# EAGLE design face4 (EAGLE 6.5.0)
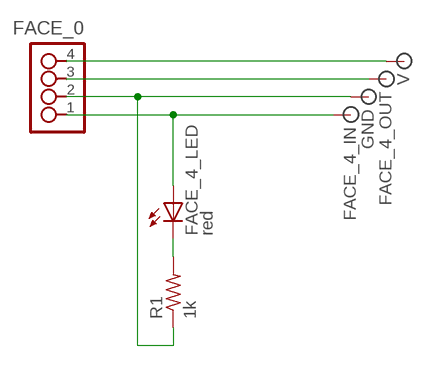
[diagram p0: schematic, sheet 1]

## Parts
FACE_0  4_PIN_HEADER  [SMT_PINS_4]
FACE_4_IN  SIGNAL  [PAD.2]
FACE_4_LED  red  LED1206  [1206]
FACE_4_OUT  SIGNAL  [PAD.2]
GND  SIGNAL  [PAD.2]
R1  1k  RESISTOR1206  [1206]
V  SIGNAL  [PAD.2]

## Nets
N$1: FACE_0.2 GND.P$1 R1.1
N$2: FACE_0.1 FACE_4_IN.P$1 FACE_4_LED.1(A)
N$4: FACE_0.3 FACE_4_OUT.P$1
N$5: FACE_4_LED.2(C) R1.2
N$6: FACE_0.4 V.P$1

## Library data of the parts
FACE_0 = ot:4_PIN_HEADER
FACE_4_IN FACE_4_OUT GND V = ot:SIGNAL: Signal
FACE_4_LED = 01_FAB_Hello:LED
R1 = 01_FAB_Hello:RESISTOR

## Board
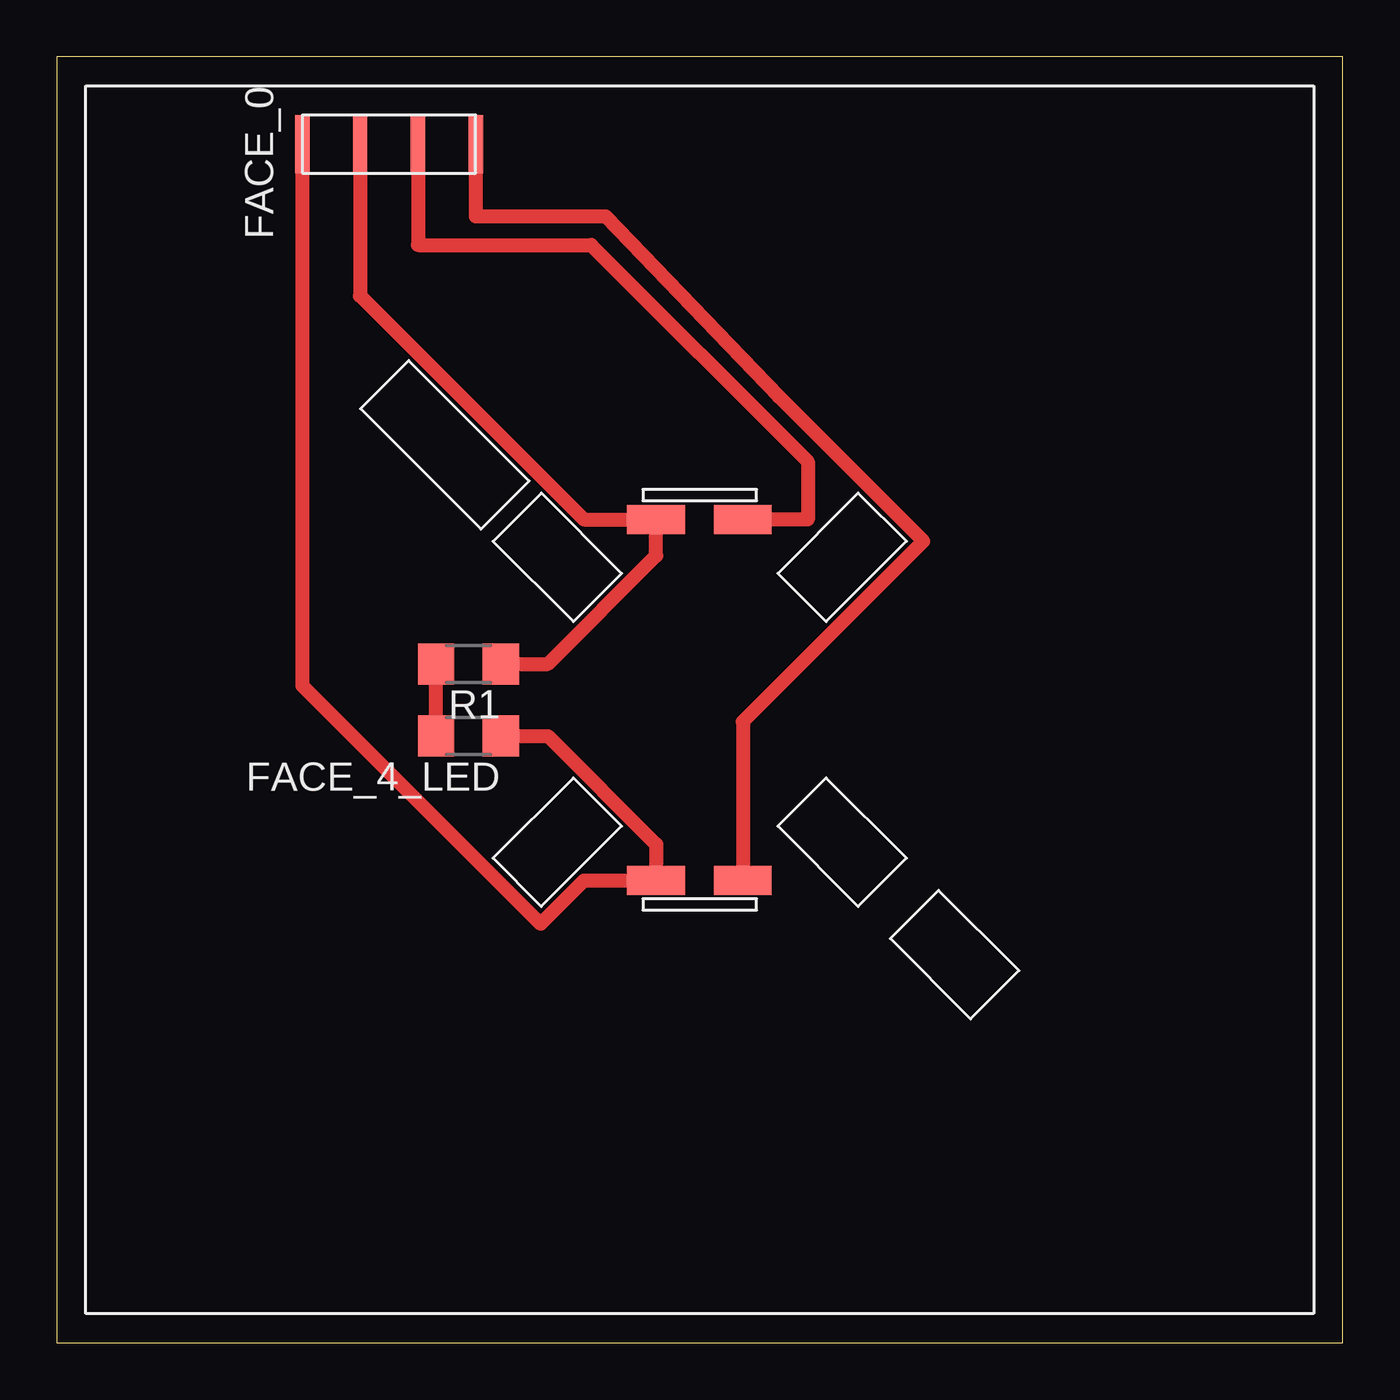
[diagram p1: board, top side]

Size 56.54 x 56.54 mm. Coordinates in mm from the lower left corner, seen from the top.
Outline: 0,0 56.54,0 56.54,56.54 0,56.54 0,0
Copper layers (1*16): Top 0.035mm / dielectric 1.5mm / Bottom 0.035mm
Design rules "default": minimum track width 10mil, minimum drill 24mil, track to track 8mil, track to pad 8mil, pad to pad 8mil, via to via 8mil, smd to smd 8mil, copper to edge 40mil, drill to drill 8mil, minimum pad ring 10mil, minimum via ring 8mil, stop-mask expansion 4mil, vias tented up to drill 0mil, thermal gap 10mil

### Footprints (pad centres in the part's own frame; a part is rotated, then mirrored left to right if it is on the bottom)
SMT_PINS_4 = smd 2.54 x 0.635: 1 0,0; 2 0,2.54; 3 0,5.08; 4 0,7.62
PAD.2 = smd 2.54 x 1.27: P$1 0,0
1206 = smd 1.6 x 1.803: 1 -1.422,0; 2 1.422,0

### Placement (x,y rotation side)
FACE_0  10.79,52.7 270 top
FACE_4_IN  26.35,20.32 0 top
FACE_4_LED  18.1,26.67 180 top
FACE_4_OUT  30.16,36.2 0 top
GND  26.35,36.2 180 top
R1  18.1,29.84 180 top
U$1  [CUBE_NEG]  55.27,1.27 90 top
V  30.16,20.32 180 top

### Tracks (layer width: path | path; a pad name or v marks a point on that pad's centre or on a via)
N$1
  Top 0.61: FACE_0.2 13.34,46.04 23.18,36.2 GND.P$1 26.35,34.61 21.59,29.84 R1.1
N$2
  Top 0.61: FACE_0.1 10.79,28.89 21.27,18.41 23.18,20.32 FACE_4_IN.P$1 26.35,21.91 21.59,26.67 FACE_4_LED.1
N$4
  Top 0.61: FACE_0.3 15.88,48.26 23.5,48.26 33.02,38.73 33.02,36.2 FACE_4_OUT.P$1
N$5
  Top 0.61: FACE_4_LED.2 R1.2
N$6
  Top 0.61: FACE_0.4 18.41,49.53 24.13,49.53 31.75,41.59 38.1,35.24 30.16,27.3 V.P$1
